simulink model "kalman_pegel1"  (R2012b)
settings: Solver=ode45  StartTime=0.0  StopTime=10.0  RelTol=1e-3
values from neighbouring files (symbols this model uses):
  Kest = kalman(P,1,0.01),    [LQG_1.m]    (also in ss_zwei_eing_1.m = kalman(sys2, Q, R))
  kp = 0.5    [kalman_pegel_1.m]
  my_sys11 = ss(my_sys11.a,my_sys11.b,eye(2,2),[0;0])    [kalman_d2.m]    (also in kalman_d3.m = ss(my_sys3.a, my_sys3.b(:,1), eye(2,2), 0); kalman_pegel_1.m = c2d(my_sys1,Ts,'zoh'))
  Ts = 0.001    [fuellstnd_3.m]    (also in fuellstnd_31.m; kalman_d1.m = 0.05; kalman_d2.m = 0.1; kalman_d3.m = 0.1)
  vnd = 1e-4    (= 0.0001)    [kalman_1.m]    (also in kalman_10.m; kalman_11.m; kalman_12.m; kalman_13.m = 0.01)
  vny = 1e-6    (= 1e-06)    [kalman_1.m]    (also in kalman_10.m; kalman_11.m = ', num2str(vny),' )']); kalman_12.m = ', num2str(vny),' )']); kalman_13.m = ', num2str(vny),' )']))
libraries: simulink x2

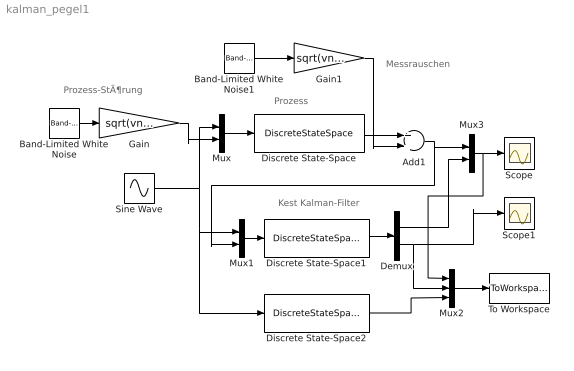
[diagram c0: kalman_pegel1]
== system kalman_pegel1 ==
  note: Messrauschen
  note: Prozess-StÃ¶rung
  note: Prozess
  note: Kest Kalman-Filter
  Add1 : Sum
  Band-Limited White Noise : simulink/Sources/Band-Limited White Noise  Cov=[Ts]  Ts=Ts  seed=[23341]
  Band-Limited White Noise1 : simulink/Sources/Band-Limited White Noise  Cov=[Ts]  Ts=Ts  seed=[267185]
  Demux : Demux  Outputs=2
  Discrete State-Space : DiscreteStateSpace  A=my_sys11.a  B=my_sys11.b  C=my_sys11.c  D=my_sys11.d  SampleTime=Ts
  Discrete State-Space1 : DiscreteStateSpace  A=Kest.a  B=Kest.b  C=Kest.c  D=Kest.d  SampleTime=Ts
  Discrete State-Space2 : DiscreteStateSpace  B=Ts*kp  D=0  SampleTime=Ts
  Gain : Gain  Gain=sqrt(vnd)*0
  Gain1 : Gain  Gain=sqrt(vny)
  Mux : Mux  Inputs=2
  Mux1 : Mux  Inputs=2
  Mux2 : Mux  Inputs=3
  Mux3 : Mux  Inputs=2
  Scope : Scope
  Scope1 : Scope
  Sine Wave : Sin  Amplitude=0.5  Bias=0.5  SampleTime=Ts
  To Workspace : ToWorkspace  VariableName=y  SampleTime=-1  SaveFormat=Structure With Time
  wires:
  Band-Limited White Noise1/1 -> Gain1/1
  Band-Limited White Noise/1 -> Gain/1
  Gain/1 -> Mux/2
  Mux/1 -> Discrete State-Space/1
  Sine Wave/1 -> Mux/1, Discrete State-Space2/1, Mux1/1
  Mux1/1 -> Discrete State-Space1/1
  Discrete State-Space/1 -> Add1/1
  Gain1/1 -> Add1/2
  Add1/1 -> Mux3/1, Mux1/2
  Discrete State-Space1/1 -> Demux/1
  Demux/1 -> Mux3/2
  Mux3/1 -> Mux2/1, Scope/1
  Demux/2 -> Mux2/2, Scope1/1
  Mux2/1 -> To Workspace/1
  Discrete State-Space2/1 -> Mux2/3
